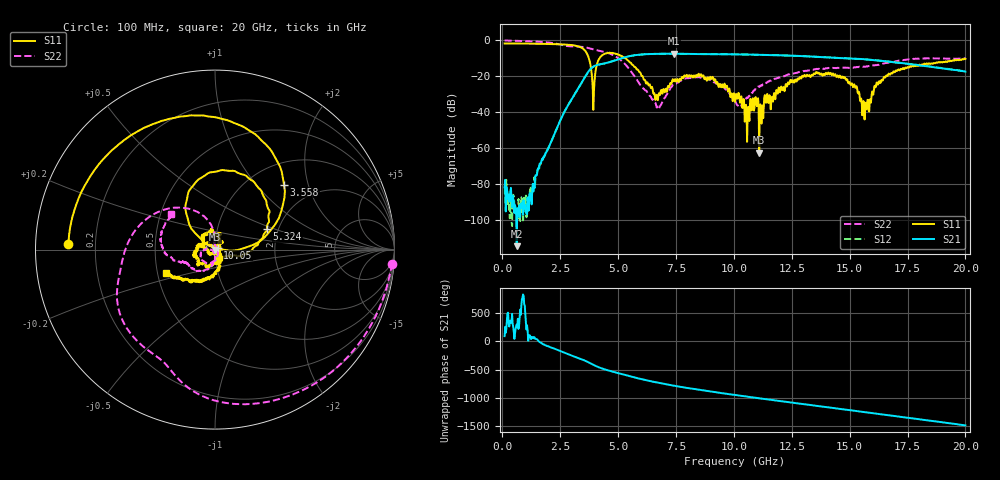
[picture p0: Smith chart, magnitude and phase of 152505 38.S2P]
!  2-Port S-parameters saved by WinCal
! VAR MeasName=S-Parameters (CALIBRATED_DATA) read from VNA (N5230C)
! VAR MeasDate=4/10/2015 9:32:16 AM
! VAR NAME=152505 38
! VAR FILENAME=152505 38.S2P
! VAR DATE=4/10/2015 9:32:16 AM
! VAR PHYS_PORTS=1,2
# Hz S DB R 50
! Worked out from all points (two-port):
!   801 points, 100 MHz to 20 GHz, reference 50 ohm
!   highest |S21| = -7.45 dB at 7.413 GHz (marker M1); lowest = -114.4 dB at 622.4 MHz (marker M2)
!   |S21| within 3 dB of the highest: 5.025 GHz to 15.57 GHz (10.54 GHz wide, 102 % of centre)
!   lowest |S11| = -62.5 dB at 11.09 GHz (marker M3), VSWR 1.00, Z = 50.1 - j0.0399 ohm
!   |S11| at or under -10 dB: 3.737 GHz to 4.2 GHz (462.4 MHz wide, 11.7 % of centre); 5.298 GHz to end of sweep
!   |S22| runs from -38.1 to -0.1 dB; largest |S21 - S12| = 0.0057
!   S11 on the Smith chart (normalised r, x): 100 MHz: 0.10, +0.02; 3.558 GHz: 1.41, +1.42; 5.324 GHz: 1.75, +0.44; 10.05 GHz: 1.03, +0.02; 20 GHz: 0.55, -0.16
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1e8  -1.75 177.6  -81.61 93.0  -81.71 44.0  -0.08 -4.6
6.22375e8  -1.78 165.1  -114.44 -63.5  -95.51 -3.2  -0.30 -25.3
1.318875e9  -1.89 147.8  -79.82 56.0  -83.68 73.3  -0.62 -53.4
2.761625e9  -2.38 101.1  -37.83 145.9  -37.86 146.0  -3.13 -112.8
3.43325e9  -4.20 57.6  -23.43 43.1  -23.42 43.4  -3.64 -138.5
3.557625e9  -5.54 43.3  -20.69 22.6  -20.68 22.8  -3.85 -144.9
3.93075e9  -38.64 53.4  -14.63 -52.9  -14.63 -52.7  -5.05 -163.5
4.32875e9  -8.15 105.8  -13.08 -120.7  -13.07 -121.1  -6.16 177.3
5.32375e9  -10.14 21.2  -9.33 124.7  -9.32 124.8  -13.53 111.2
6.741625e9  -30.54 -131.0  -7.50 -10.6  -7.49 -10.8  -37.61 29.9
7.41325e9  -22.84 164.9  -7.45 -61.7  -7.46 -61.8  -24.62 -86.1
8.90575e9  -21.01 82.1  -7.71 -159.3  -7.73 -159.1  -21.69 -165.2
1.005e10  -34.23 36.9  -7.80 133.9  -7.82 133.9  -33.95 -173.7
1.057238e10  -56.43 121.0  -7.93 104.5  -7.92 104.3  -31.94 -93.6
1.092062e10  -32.00 29.4  -8.03 85.4  -8.04 85.7  -27.39 -88.4
1.109475e10  -62.47 -31.9  -8.08 75.9  -8.05 75.6  -25.95 -89.1
1.141812e10  -30.91 -14.7  -8.18 58.2  -8.19 58.3  -23.63 -93.6
1.338325e10  -19.28 -129.8  -9.06 -46.8  -9.02 -46.6  -16.31 -128.1
1.480112e10  -20.65 164.1  -9.98 -120.4  -9.99 -121.2  -15.18 -153.4
1.564688e10  -43.99 50.6  -10.57 -166.9  -10.61 -166.0  -14.68 -156.1
1.669162e10  -18.50 -79.9  -11.84 136.7  -11.80 136.5  -12.40 -166.1
2e10  -10.34 -154.2  -17.37 -43.2  -17.30 -43.2  -10.06 140.5
